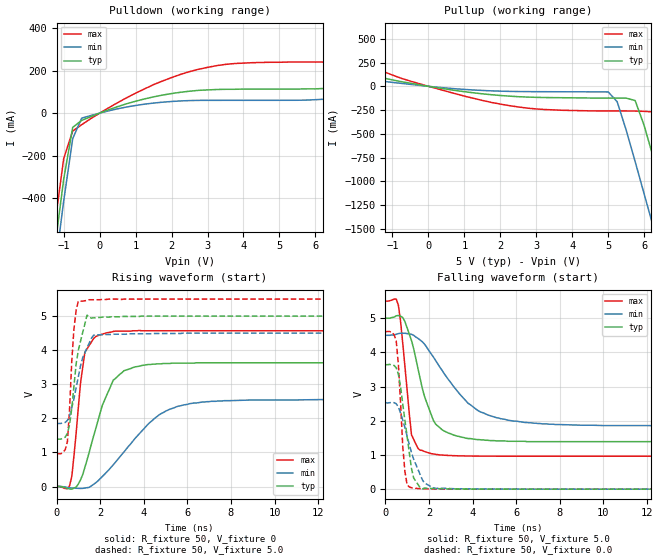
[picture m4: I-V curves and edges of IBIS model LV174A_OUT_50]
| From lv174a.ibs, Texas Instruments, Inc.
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|   Model LV174A_OUT_50
[Model]   LV174A_OUT_50
Model_type  Output
Polarity   Non-Inverting
Vmeas = 2.50v
Cref = 15pf
| variable   typ   min   max
C_comp   5.60pf   4.20pf   7.00pf
[Temperature Range]   25   85   -40
[Voltage Range]   5.0   4.5   5.5
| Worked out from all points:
|   slope of the pulldown table from 0 to 0.75 V, typ, clamps not added: 17 ohm
|   slope of the pullup table from 0 to 0.75 V, typ, clamps not added: 17.2 ohm
|   rising waveform, R_fixture 50, V_fixture 0: 20-80 % time 1.08ns typ, 2.15ns min, 435ps max; typ from 0 V to 3.63 V
|   falling waveform, R_fixture 50, V_fixture 5.0: 20-80 % time 916ps typ, 1.99ns min, 405ps max; typ from 5 V to 1.39 V
|   rising waveform, R_fixture 50, V_fixture 5.0: 20-80 % time 446ps typ, 607ps min, 240ps max; typ from 1.39 V to 5 V
|   falling waveform, R_fixture 50, V_fixture 0.0: 20-80 % time 458ps typ, 748ps min, 251ps max; typ from 3.64 V to 0 V
[Pulldown]
|   Voltage   I(typ)   I(min)   I(max)
-5V       -5.91A     -6A        -5.81A
-1.25V    -636mA     -741mA     -527mA
-1V       -310mA     -412mA     -213mA
-750mV    -67mA      -120mA     -84.1mA
-500mV    -34.1mA    -23.4mA    -54.3mA
0V        -3.33nA    -3.4nA     -3.57nA
1.5V      76.4mA     47.3mA     134mA
2.75V     107mA      59.9mA     206mA
3.75V     112mA      60.2mA     233mA
7V        129mA      75.3mA     253mA
8.25V     162mA      97.9mA     302mA
10V       222mA      135mA      404mA
[Pullup]
|   Voltage   I(typ)   I(min)   I(max)
-5V       328mA      183mA      611mA
1.5V      -78.8mA    -43.5mA    -148mA
3V        -116mA     -56.1mA    -238mA
5V        -123mA     -58.9mA    -259mA
5.25V     -123mA     -162mA     -259mA
5.75V     -149mA     -790mA     -260mA
6.25V     -740mA     -1.47A     -269mA
6.5V      -1.08A     -1.82A     -421mA
6.75V     -1.43A     -2.17A     -745mA
7.25V     -2.13A     -2.87A     -1.43A
7.5V      -2.48A     -3.23A     -1.78A
10V       -6.01A     -6.76A     -5.32A
[Ramp]
| variable   typ   min   max
dV/dt_r   2.18E+00/1.05E-09   1.54E+00/2.15E-09   2.78E+00/4.35E-10
dV/dt_f   2.22E+00/8.84E-10   1.63E+00/1.98E-09   2.77E+00/4.16E-10
R_load = 50
[Rising Waveform]
R_fixture = 50
V_fixture = 0
|   Time   V(typ)   V(min)   V(max)
0s        0V         0V         0V
500ps     -55.6mV    -30mV      -65.3mV
700ps     -77.6mV    -44.8mV    296mV
1.1ns     195mV      -57mV      3.03V
1.3ns     562mV      -44.2mV    3.94V
2.3ns     2.68V      423mV      4.51V
3.1ns     3.4V       1.02V      4.56V
4.7ns     3.6V       2.1V       4.57V
6.3ns     3.62V      2.45V      4.57V
25ns      3.63V      2.55V      4.57V
[Falling Waveform]
R_fixture = 50
V_fixture = 5.0
V_fixture_min = 4.5
V_fixture_max = 5.5
|   Time   V(typ)   V(min)   V(max)
0s        5V         4.5V       5.5V
600ps     5.08V      4.55V      5.38V
900ps     4.9V       4.56V      3.59V
1.2ns     4.35V      4.53V      1.59V
1.5ns     3.52V      4.41V      1.19V
2.1ns     2.19V      3.96V      1.04V
2.6ns     1.74V      3.48V      999mV
3.8ns     1.48V      2.51V      969mV
5.9ns     1.4V       1.99V      964mV
25ns      1.39V      1.85V      963mV
[Rising Waveform]
R_fixture = 50
V_fixture = 5.0
V_fixture_min = 4.5
V_fixture_max = 5.5
|   Time   V(typ)   V(min)   V(max)
0s        1.39V      1.85V      963mV
400ps     1.45V      1.88V      1.08V
500ps     1.56V      1.94V      1.32V
600ps     1.82V      2.07V      2.3V
700ps     2.3V       2.31V      3.69V
800ps     2.95V      2.58V      4.63V
1ns       4V         3.22V      5.44V
1.4ns     5.03V      4.07V      5.46V
1.7ns     4.95V      4.44V      5.48V
25ns      5V         4.5V       5.5V
[Falling Waveform]
R_fixture = 50
V_fixture = 0.0
|   Time   V(typ)   V(min)   V(max)
0s        3.64V      2.53V      4.61V
500ps     3.55V      2.5V       4.34V
600ps     3.36V      2.4V       3.64V
800ps     2.49V      2.02V      1.25V
900ps     2.01V      1.8V       508mV
1ns       1.54V      1.55V      129mV
1.2ns     608mV      1.07V      41.2mV
1.6ns     42.1mV     424mV      15.8mV
2.3ns     16.6mV     21.9mV     5.58mV
25ns      0V         0V         6.99uV
